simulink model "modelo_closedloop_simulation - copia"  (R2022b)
settings: Solver=ode45  StartTime=0.0  StopTime=1  MaxStep=1e-6  RelTol=1e-3
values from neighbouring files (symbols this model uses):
  fsw = 36e3    (= 36000)    [closedloop_analysis - copia.m]
  ki = wc*R    (= 20)    [closedloop_analysis - copia.m]
  kp = wc*L    (= 0.2)    [closedloop_analysis - copia.m]
  L = 100e-6    (= 0.0001)    [closedloop_analysis - copia.m]
  R = 0.01    [closedloop_analysis - copia.m]
  Ts = Tsw    (= 2.77777777778e-05)    [closedloop_analysis - copia.m]
  Tsim = Tsw/400    (= 6.94444444444e-08)    [closedloop_analysis - copia.m]
  Vdc = 450    [closedloop_analysis - copia.m]
undefined symbols (not defined in the file or in its folder): arm, bridge, pulses
libraries: simulink x12, spsMosfetLib x6, spsCurrentMeasurementLib x3, spsSeriesRLCBranchLib x3, powerlib_extras x3, slpidlib x2, spsControlledVoltageSourceLib x1, spsGroundLib x1, spsDCVoltageSourceLib x1, sps_lib x1

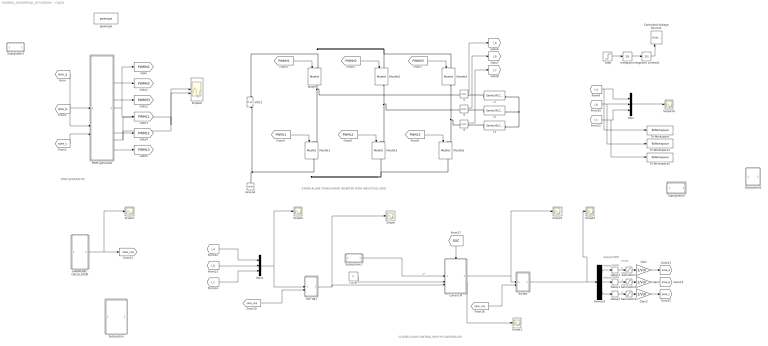
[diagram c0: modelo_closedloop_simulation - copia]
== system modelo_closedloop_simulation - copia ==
  note: CLOSED LOOP CONTROL WITH PI CONTROLLER
  note: STAND ALONE THREE-PHASE INVERTER WITH INDUCTIVE LOAD
  note: PWM GENERATOR
  note: vmax
  note: reload PWM
  note: vmax
  note: reload PWM
  note: reload PWM
  note: vmax
  Controlled Voltage Source1 : spsControlledVoltageSourceLib/Controlled Voltage Source  Commented=on  Initialize=on  Source_Type=AC  Amplitude=0  Phase=0  Frequency=0  Measurements=None
  Delay1 : Delay  DelayLength=1  SampleTime=Ts/2
  Delay2 : Delay  DelayLength=1  SampleTime=Ts/2
  Delay3 : Delay  DelayLength=1  SampleTime=Ts/2
  Demux5 : Demux  Outputs=3
  Gain : Gain  Gain=1/Vdc
  Gain1 : Gain  Gain=1/Vdc
  Gain2 : Gain  Gain=1/Vdc
  Ground : spsGroundLib/Ground  LConnTagsString=a
  HARMONIC OSCILLATOR : Subsystem
  I1 : spsCurrentMeasurementLib/Current Measurement  PhasorSimulation=off  OutputType=Complex  PSBequivalent=0
  I2 : spsCurrentMeasurementLib/Current Measurement  PhasorSimulation=off  OutputType=Complex  PSBequivalent=0
  I3 : spsCurrentMeasurementLib/Current Measurement  PhasorSimulation=off  OutputType=Complex  PSBequivalent=0
  Integrator : Integrator  Commented=on
  Integrator Limited1 : Integrator  Commented=on  LimitOutput=on  UpperSaturationLimit=900  LowerSaturationLimit=0
  L1 : spsSeriesRLCBranchLib/Series RLC Branch  LConnTagsString=__new0  RConnTagsString=__new0  BranchType=RL  Resistance=R  Inductance=L  SetiL0=off  InitialCurrent=0  Capacitance=1e-6  Setx0=off  InitialVoltage=0  Measurements=None
  L2 : spsSeriesRLCBranchLib/Series RLC Branch  LConnTagsString=__new0  RConnTagsString=__new0  BranchType=RL  Resistance=R  Inductance=L  SetiL0=off  InitialCurrent=0  Capacitance=1e-6  Setx0=off  InitialVoltage=0  Measurements=None
  L3 : spsSeriesRLCBranchLib/Series RLC Branch  LConnTagsString=__new0  RConnTagsString=__new0  BranchType=RL  Resistance=R  Inductance=L  SetiL0=off  InitialCurrent=0  Capacitance=1e-6  Setx0=off  InitialVoltage=0  Measurements=None
  Mosfet{,1..5} (6 alike) : spsMosfetLib/Mosfet  Ron=0.1  Lon=0  Rd=0.01  Vfd=1  IC=0  Rs=1e5  Cs=inf  Measurements=off
  Mux : Mux  Inputs=3
  Mux1 : Mux  Inputs=3
  PWM generator : Subsystem
  Saturation : Saturate  UpperLimit=Vdc*0.98  LowerLimit=0
  Saturation1 : Saturate  UpperLimit=Vdc*0.98  LowerLimit=0
  Saturation2 : Saturate  UpperLimit=Vdc*0.98  LowerLimit=0
  Scope{,1..3,5,7,10} (7 alike) : Scope
  Scope9 : Scope  NumInputPorts=2
  Step : Step  Commented=on  Time=0  After=2500  SampleTime=0
  Subsystem : Subsystem  Commented=on
  Subsystem1 : Subsystem
  Subsystem2 : Subsystem  Commented=on
  Subsystem3 : Subsystem  Commented=on
  Subsystem4 : Subsystem
  To Workspace : ToWorkspace  VariableName=i_a  SaveFormat=Structure With Time  SampleTime=-1
  To Workspace1 : ToWorkspace  VariableName=i_b  SaveFormat=Structure With Time  SampleTime=-1
  To Workspace2 : ToWorkspace  VariableName=i_c  SaveFormat=Structure With Time  SampleTime=-1
  VDC1 : spsDCVoltageSourceLib/DC Voltage Source  Amplitude=Vdc*2  Measurements=None
  abc-dq1 : Subsystem
  current PI : Subsystem
  dq-abc : Subsystem
  i_q ref : Constant  Value=0
  powergui : sps_lib/powergui  Priority=1  SimulationMode=Continuous  SampleTime=50e-6  frequency=60  Iterations=50  frequencyindice=0  Pbase=100e6  ErrMax=1e-4  UnitsV=kV  UnitsW=MW  buscounter=0  FunctionMessages=off  echomessages=off  EnableUseOfTLC=off  CurrentSourceSwitches=off  DisableSnubberDevices=off  DisableRonSwitches=off  DisableVfSwitches=off  DisplayEquations=off  AutomaticDiscreteSolvers=off  SolverType=Tustin/Backward Euler (TBE)  Interpol=off  ExternalGateDelay=off  methode=off  Ts=100  x0status=blocks  SPID=on  SwTol=0  HookPort=off  NonlinearTolerance=1e-4  nMaxIteration=100  ContinueOnMaxIteration=off  RestoreLinks=warning  ResistiveCurrentMeasurement=off  Frange=[0:2:500]  Ylog=off  Xlog=on  ShowGrid=off  save=off  variable=ZData  structure=0  ZoomFFT=off  StartTime=0.0  cycles=1  DisplayStyle=1  fundamental=60  FreqAxis=off  MaxFrequency=1000  frequencyindicesteady=1  RmsSteady=1  display=off
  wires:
  [sine_a] -> PWM generator/1(m1)
  [sine_b] -> PWM generator/2(m2)
  [sine_c] -> PWM generator/3(m3)
  PWM generator/1(PWMH1) -> Scope9/1, [PWMH1]
  PWM generator/2(PWMH2) -> [PWMH2]
  PWM generator/3(PWMH3) -> [PWMH3]
  PWM generator/4(PWML1) -> Scope9/2, [PWML1]
  PWM generator/5(PWML2) -> [PWML2]
  PWM generator/6(PWML3) -> [PWML3]
  [PWMH1] -> Mosfet/1
  [PWML1] -> Mosfet1/1
  [PWML2] -> Mosfet3/1
  [PWMH2] -> Mosfet2/1
  [PWML3] -> Mosfet5/1
  [PWMH3] -> Mosfet4/1
  I1/1 -> [i_a]
  I2/1 -> [i_b]
  I3/1 -> [i_c]
  HARMONIC OSCILLATOR/1(sin-cos) -> Scope7/1, [sine_cos]
  [i_c] -> Mux1/3
  [i_b] -> Mux1/2
  [i_a] -> Mux1/1
  Mux1/1 -> Scope5/1, abc-dq1/1(abc)
  [sine_cos] -> abc-dq1/2(sin-cos)
  abc-dq1/1(dq) -> Scope/1, current PI/3(dq pi in)
  [sine_cos] -> dq-abc/2(sin-cos)
  Step/1 -> Integrator/1
  Integrator/1 -> Integrator Limited1/1
  Integrator Limited1/1 -> Controlled Voltage Source1/1
  dq-abc/1(abc) -> Scope3/1, Demux5/1
  current PI/1(dq pi out) -> dq-abc/1(dq), Scope2/1
  [i_a] -> To Workspace/1, Mux/1
  [i_b] -> To Workspace1/1, Mux/2
  [i_c] -> To Workspace2/1, Mux/3
  Mux/1 -> Scope10/1
  i_q ref/1 -> current PI/2(q ref)
  Subsystem1/1(y*) -> current PI/1(d ref)  "y*"
  Delay3/1 -> Saturation/1  "u"
  Saturation/1 -> Gain/1
  Delay1/1 -> Saturation1/1  "u"
  Saturation1/1 -> Gain1/1
  Delay2/1 -> Saturation2/1  "u"
  Saturation2/1 -> Gain2/1
  Demux5/3 -> Delay2/1
  Demux5/2 -> Delay1/1
  Demux5/1 -> Delay3/1
  Gain/1 -> [sine_a]
  Gain1/1 -> [sine_b]
  Gain2/1 -> [sine_c]
  [SOC] -> current PI/Trigger
  current PI/2(debug) -> Scope1/1
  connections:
  Mosfet/RConn1 -- I1/LConn1 -- Mosfet1/LConn1
  Mosfet2/RConn1 -- I2/LConn1 -- Mosfet3/LConn1
  L3/LConn1 -- I3/RConn1
  VDC1/RConn1 -- Mosfet4/LConn1 -- Mosfet2/LConn1 -- Mosfet/LConn1
  Mosfet1/RConn1 -- Mosfet3/RConn1 -- Mosfet5/RConn1 -- Ground/LConn1 -- VDC1/LConn1
  L1/RConn1 -- L2/RConn1 -- L3/RConn1
  L1/LConn1 -- I1/RConn1
  L2/LConn1 -- I2/RConn1
  Mosfet4/RConn1 -- I3/LConn1 -- Mosfet5/LConn1

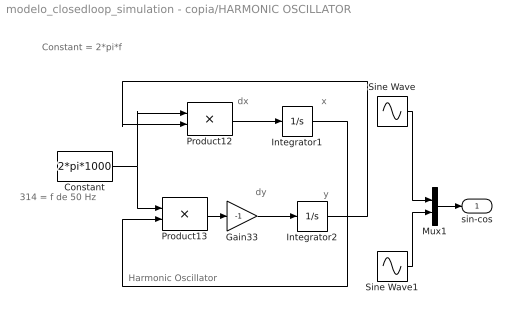
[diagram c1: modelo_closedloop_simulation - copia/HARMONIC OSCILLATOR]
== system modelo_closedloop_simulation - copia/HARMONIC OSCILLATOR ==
  note: 314 = f de 50 Hz
  note: Constant = 2*pi*f
  note: Harmonic Oscillator
  note: dy
  note: dx
  note: y
  note: x
  Constant : Constant  Commented=on  Value=2*pi*1000
  Gain33 : Gain  Commented=on  Gain=-1  SaturateOnIntegerOverflow=on
  Integrator1 : Integrator  Commented=on  InitialCondition=1  LimitOutput=on  UpperSaturationLimit=1  LowerSaturationLimit=-1
  Integrator2 : Integrator  Commented=on  LimitOutput=on  UpperSaturationLimit=1  LowerSaturationLimit=-1
  Mux1 : Mux  Inputs=2
  Product12 : Product  Commented=on  SaturateOnIntegerOverflow=on
  Product13 : Product  Commented=on  SaturateOnIntegerOverflow=on
  Sine Wave : Sin  SineType=Sample based  Samples=fsw/1000  SampleTime=Ts
  Sine Wave1 : Sin  SineType=Sample based  Samples=fsw/1000  SampleTime=Ts
  sin-cos : Outport  VectorParamsAs1DForOutWhenUnconnected=off
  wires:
  Constant/1 -> Product13/1, Product12/1
  Gain33/1 -> Integrator2/1
  Product12/1 -> Integrator1/1
  Product13/1 -> Gain33/1
  Integrator1/1 -> Product13/2
  Integrator2/1 -> Product12/2
  Mux1/1 -> sin-cos/1
  Sine Wave1/1 -> Mux1/2
  Sine Wave/1 -> Mux1/1

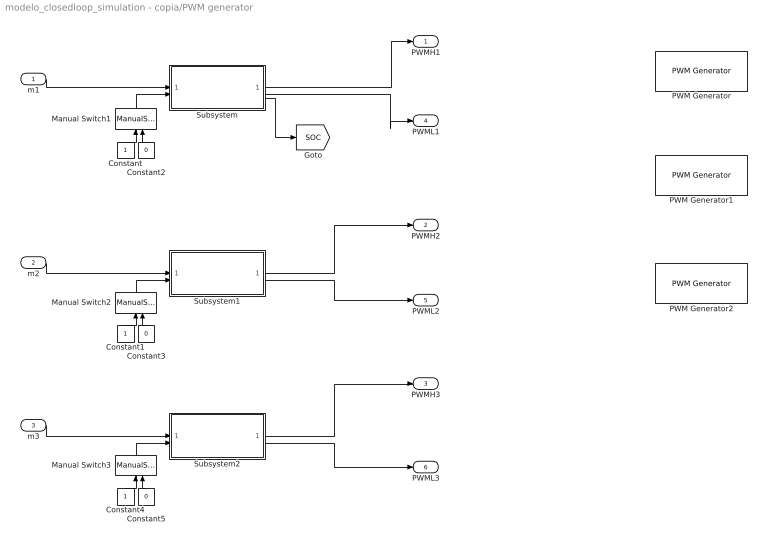
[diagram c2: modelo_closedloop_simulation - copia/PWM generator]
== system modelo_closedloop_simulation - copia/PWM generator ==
  m1 : Inport
  m2 : Inport  Port=2
  m3 : Inport  Port=3
  Constant : Constant  SampleTime=Ts
  Constant1 : Constant  SampleTime=Ts
  Constant2 : Constant  Value=0  SampleTime=Ts
  Constant3 : Constant  Value=0  SampleTime=Ts
  Constant4 : Constant  SampleTime=Ts
  Constant5 : Constant  Value=0  SampleTime=Ts
  Manual Switch1 : ManualSwitch
  Manual Switch2 : ManualSwitch
  Manual Switch3 : ManualSwitch
  PWM Generator : powerlib_extras/Control  Blocks/PWM Generator  Commented=on  GeneratorMode="1-arm  bridge (2 pulses)"  Fc=36e3  Internal=off  mIndex=0.4  Freq=60  Phase=0
  PWM Generator1 : powerlib_extras/Control  Blocks/PWM Generator  Commented=on  GeneratorMode="1-arm  bridge (2 pulses)"  Fc=36e3  Internal=off  mIndex=0.4  Freq=60  Phase=0
  PWM Generator2 : powerlib_extras/Control  Blocks/PWM Generator  Commented=on  GeneratorMode="1-arm  bridge (2 pulses)"  Fc=36e3  Internal=off  mIndex=0.4  Freq=60  Phase=0
  Subsystem : Subsystem
  Subsystem1 : Subsystem
  Subsystem2 : Subsystem
  PWMH1 : Outport  VectorParamsAs1DForOutWhenUnconnected=off
  PWMH2 : Outport  Port=2  VectorParamsAs1DForOutWhenUnconnected=off
  PWMH3 : Outport  Port=3  VectorParamsAs1DForOutWhenUnconnected=off
  PWML1 : Outport  Port=4  VectorParamsAs1DForOutWhenUnconnected=off
  PWML2 : Outport  Port=5  VectorParamsAs1DForOutWhenUnconnected=off
  PWML3 : Outport  Port=6  VectorParamsAs1DForOutWhenUnconnected=off
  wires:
  Subsystem1/2(s1B) -> PWML2/1
  Subsystem/2(s1B) -> PWML1/1
  Subsystem/1(s1A) -> PWMH1/1
  Subsystem/3(SOC) -> [SOC]
  m1/1 -> Subsystem/1(modA)
  Constant/1 -> Manual Switch1/1
  Constant2/1 -> Manual Switch1/2
  Manual Switch1/1 -> Subsystem/2(enable delay)
  Manual Switch2/1 -> Subsystem1/2(enable delay)
  Constant3/1 -> Manual Switch2/2
  Constant1/1 -> Manual Switch2/1
  m2/1 -> Subsystem1/1(modA)
  Subsystem1/1(s1A) -> PWMH2/1
  Manual Switch3/1 -> Subsystem2/2(enable delay)
  Constant5/1 -> Manual Switch3/2
  Subsystem2/2(s1B) -> PWML3/1
  Constant4/1 -> Manual Switch3/1
  m3/1 -> Subsystem2/1(modA)
  Subsystem2/1(s1A) -> PWMH3/1

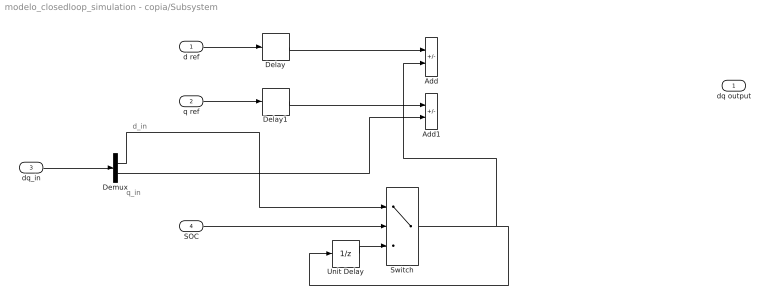
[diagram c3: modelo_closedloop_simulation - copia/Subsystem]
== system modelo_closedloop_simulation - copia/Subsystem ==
  note: q_in
  note: d_in
  d ref : Inport
  q ref : Inport  Port=2
  dq_in : Inport  Port=3
  SOC : Inport  Port=4
  Add : Sum  Inputs=+-
  Add1 : Sum  Inputs=+-
  Delay : Delay  DelayLength=1  SampleTime=Ts/2
  Delay1 : Delay  DelayLength=1  SampleTime=Ts/2
  Demux : Demux  Outputs=2
  Switch : Switch
  Unit Delay : UnitDelay  SampleTime=-1  HasFrameUpgradeWarning=on
  dq output : Outport
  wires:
  d ref/1 -> Delay/1
  q ref/1 -> Delay1/1
  dq_in/1 -> Demux/1
  Demux/1 -> Switch/1
  Delay/1 -> Add/1
  Demux/2 -> Add1/2
  Delay1/1 -> Add1/1
  SOC/1 -> Switch/2
  Unit Delay/1 -> Switch/3
  Switch/1 -> Add/2, Unit Delay/1

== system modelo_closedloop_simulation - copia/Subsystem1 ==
  note: in practice period of 1.352s
  Add2 : Sum
  Constant : Constant  Value=127.3
  Pulse Generator : DiscretePulseGenerator  PulseType=Time based  Amplitude=6  Period=3  PulseWidth=50
  pulses : DiscretePulseGenerator  Amplitude=127.3  Period=120  PulseWidth=60  PhaseDelay=5  SampleTime=Ts
  reference step : Step  Time=2e-3  After=1.8  SampleTime=Ts
  reference step1 : Step  Time=0.01  After=-1.8  SampleTime=Ts
  y* : Outport  VectorParamsAs1DForOutWhenUnconnected=off
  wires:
  reference step1/1 -> Add2/2  "y2"
  pulses/1 -> y*/1, [iref]  "y*"
  reference step/1 -> Add2/1  "y1"

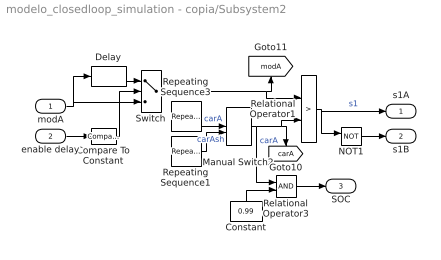
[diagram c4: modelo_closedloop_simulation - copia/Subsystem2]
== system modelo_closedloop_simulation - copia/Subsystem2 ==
  modA : Inport
  enable delay : Inport  Port=2
  Compare To Constant : simulink/Logic and Bit Operations/Compare To Constant  relop=>  const=0  OutDataTypeStr=boolean
  Constant : Constant  Value=0.99  SampleTime=Ts
  Delay : Delay  DelayLength=400  SampleTime=Tsim
  Manual Switch2 : ManualSwitch
  NOT1 : Logic  Operator=NOT  IconShape=distinctive  AllPortsSameDT=off  OutDataTypeStr=boolean
  Relational Operator1 : RelationalOperator  Operator=>  OutDataTypeStr=boolean  RndMeth=Simplest
  Relational Operator3 : RelationalOperator  OutDataTypeStr=boolean  RndMeth=Simplest
  Repeating Sequence1 : simulink/Sources/Repeating Sequence  rep_seq_t=[0 1/(4*fsw) 1/(2*fsw) 3/(4*fsw) 1/fsw]  rep_seq_y=[0.5 0 0.5 1 0.5]
  Repeating Sequence3 : simulink/Sources/Repeating Sequence  rep_seq_t=[0 1/(2*fsw) 1/fsw]  rep_seq_y=[0 1 0]
  Switch : Switch  Criteria=u2 > Threshold
  s1A : Outport  VectorParamsAs1DForOutWhenUnconnected=off
  s1B : Outport  Port=2  VectorParamsAs1DForOutWhenUnconnected=off
  SOC : Outport  Port=3  VectorParamsAs1DForOutWhenUnconnected=off
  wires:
  enable delay/1 -> Compare To Constant/1
  Relational Operator1/1 -> NOT1/1, s1A/1  "s1"
  Relational Operator3/1 -> SOC/1
  NOT1/1 -> s1B/1
  Constant/1 -> Relational Operator3/2
  Switch/1 -> Relational Operator1/1, [modA]
  modA/1 -> Delay/1, Switch/3
  Repeating Sequence1/1 -> Manual Switch2/2  "carAsh"
  Delay/1 -> Switch/1
  Manual Switch2/1 -> Relational Operator3/1, [carA], Relational Operator1/2  "carA"
  Repeating Sequence3/1 -> Manual Switch2/1  "carA"
  Compare To Constant/1 -> Switch/2

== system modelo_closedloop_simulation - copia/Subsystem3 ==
  note: in practice period of 1.352s
  Add2 : Sum
  Pulse Generator : DiscretePulseGenerator  PulseType=Time based  Amplitude=6  Period=3  PulseWidth=50
  pulses : DiscretePulseGenerator  Amplitude=1.5  Period=120  PulseWidth=60  PhaseDelay=5  SampleTime=Ts
  reference step : Step  Time=2e-3  After=1.8  SampleTime=Ts
  reference step1 : Step  Time=0.01  After=-1.8  SampleTime=Ts
  y* : Outport  VectorParamsAs1DForOutWhenUnconnected=off
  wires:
  reference step1/1 -> Add2/2  "y2"
  pulses/1 -> [iref], y*/1  "y*"
  reference step/1 -> Add2/1  "y1"

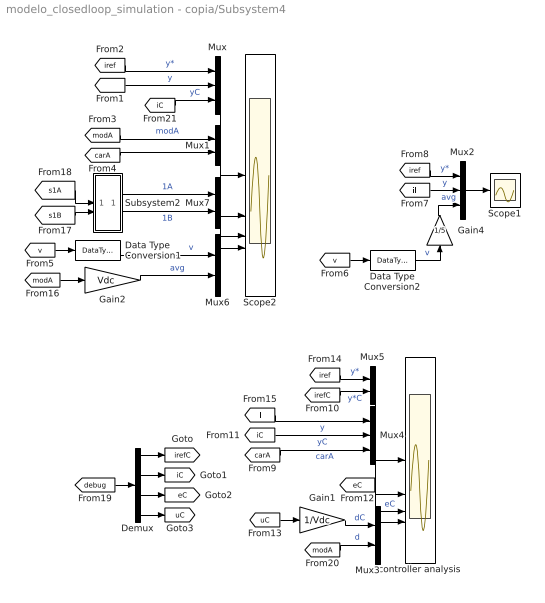
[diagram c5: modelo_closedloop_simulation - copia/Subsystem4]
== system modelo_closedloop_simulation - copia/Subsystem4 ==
  Data Type Conversion1 : DataTypeConversion  OutDataTypeStr=double
  Data Type Conversion2 : DataTypeConversion  OutDataTypeStr=double
  Demux : Demux
  Gain1 : Gain  Gain=1/Vdc
  Gain2 : Gain  Gain=Vdc
  Gain4 : Gain  Gain=1/5
  Mux : Mux  Inputs=3
  Mux{1,3,5..7} (5 alike) : Mux  Inputs=2
  Mux2 : Mux  Inputs=3
  Mux4 : Mux  Inputs=3
  Scope1 : Scope
  Scope2 : Scope  NumInputPorts=4
  Subsystem2 : Subsystem
  controller analysis : Scope  NumInputPorts=4
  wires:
  Mux1/1 -> Scope2/2
  Data Type Conversion1/1 -> Mux6/1  "v"
  [modA] -> Gain2/1
  Mux6/1 -> Scope2/4
  [carA] -> Mux1/2
  [v] -> Data Type Conversion1/1
  [s1B] -> Subsystem2/2(In2)
  Gain2/1 -> Mux6/2  "avg"
  Subsystem2/1(Out1) -> Mux7/1  "1A"
  Mux7/1 -> Scope2/3
  [modA] -> Mux1/1  "modA"
  Subsystem2/2(Out2) -> Mux7/2  "1B"
  [s1A] -> Subsystem2/1(In1)
  [v] -> Data Type Conversion2/1
  Data Type Conversion2/1 -> Gain4/1  "v"
  [iref] -> Mux2/1  "y*"
  [il] -> Mux2/2  "y"
  Mux2/1 -> Scope1/1
  Gain4/1 -> Mux2/3  "avg"
  [iref] -> Mux/1  "y*"
  [il] -> Mux/2  "y"
  Mux/1 -> Scope2/1
  [eC] -> controller analysis/3  "eC"
  Mux3/1 -> controller analysis/4
  Mux5/1 -> controller analysis/1
  Mux4/1 -> controller analysis/2
  [iref] -> Mux5/1  "y*"
  [uC] -> Gain1/1
  [il] -> Mux4/1  "y"
  [iC] -> Mux4/2  "yC"
  [carA] -> Mux4/3  "carA"
  [modA] -> Mux3/2  "d"
  [debug] -> Demux/1
  Demux/3 -> [eC]
  Demux/2 -> [iC]
  Demux/1 -> [irefC]
  Demux/4 -> [uC]
  [irefC] -> Mux5/2  "y*C"
  Gain1/1 -> Mux3/1  "dC"
  [iC] -> Mux/3  "yC"

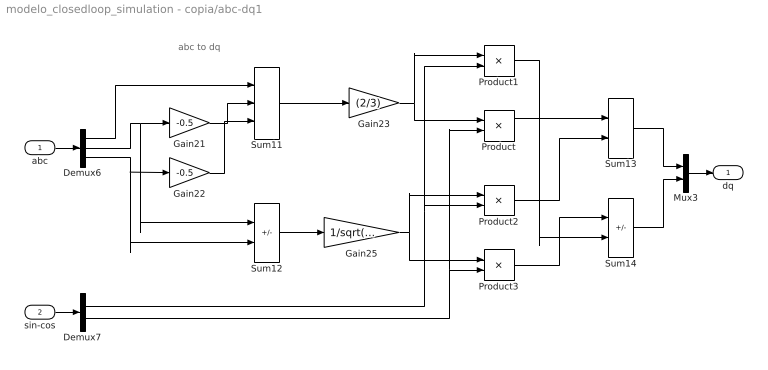
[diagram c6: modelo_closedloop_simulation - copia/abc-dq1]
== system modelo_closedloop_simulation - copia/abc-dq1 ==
  note: abc to dq
  abc : Inport
  sin-cos : Inport  Port=2
  Demux6 : Demux  Outputs=3
  Demux7 : Demux  Outputs=2
  Gain21 : Gain  Gain=-0.5
  Gain22 : Gain  Gain=-0.5
  Gain23 : Gain  Gain=(2/3)
  Gain25 : Gain  Gain=1/sqrt(3)
  Mux3 : Mux  Inputs=2
  Product{,1..3} (4 alike) : Product  RndMeth=Zero
  Sum11 : Sum  Inputs=|+++
  Sum12 : Sum  Inputs=|+-
  Sum13 : Sum  Inputs=|++
  Sum14 : Sum  Inputs=|+-
  dq : Outport  VectorParamsAs1DForOutWhenUnconnected=off
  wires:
  Sum11/1 -> Gain23/1
  Sum12/1 -> Gain25/1
  Demux6/3 -> Gain22/1, Sum12/2
  Demux6/2 -> Gain21/1, Sum12/1
  Demux6/1 -> Sum11/1
  Gain21/1 -> Sum11/2
  Gain22/1 -> Sum11/3
  Gain23/1 -> Product/1, Product1/1
  Demux7/2 -> Product/2, Product3/2
  Demux7/1 -> Product1/2, Product2/2
  Gain25/1 -> Product2/1, Product3/1
  Product/1 -> Sum13/1
  Product2/1 -> Sum13/2
  Product3/1 -> Sum14/1
  Product1/1 -> Sum14/2
  Sum13/1 -> Mux3/1
  Sum14/1 -> Mux3/2
  abc/1 -> Demux6/1
  Mux3/1 -> dq/1
  sin-cos/1 -> Demux7/1

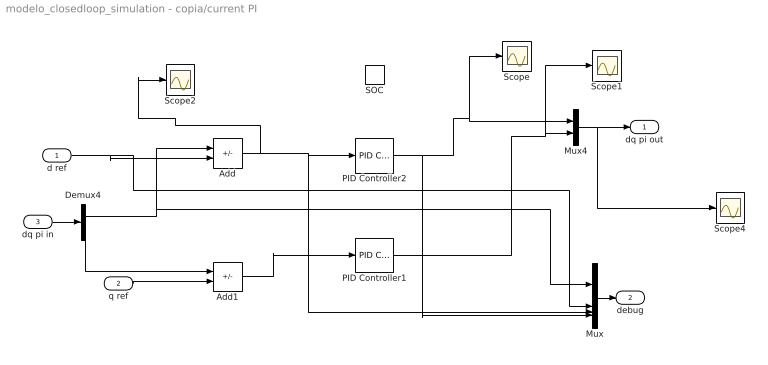
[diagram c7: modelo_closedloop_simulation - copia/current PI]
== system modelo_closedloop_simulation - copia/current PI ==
  d ref : Inport
  q ref : Inport  Port=2
  dq pi in : Inport  Port=3
  SOC : TriggerPort  VariantControl=Variant
  Add : Sum  Inputs=+-
  Add1 : Sum  Inputs=+-
  Demux4 : Demux  Outputs=2
  Mux : Mux
  Mux4 : Mux  Inputs=2
  PID Controller1 : slpidlib/PID Controller  Controller=PI  Form=Parallel  TimeDomain=Discrete-time  UseExternalTs=off  SampleTime=-1  IntegratorMethod=Backward Euler  FilterMethod=Forward Euler  ControllerParametersSource=internal  P=kp  I=ki  UseKiTs=off  D=0  N=100  UseFilter=on  TunerSelectOption=Transfer Function Based (PID Tuner App)  InitialConditionSource=internal  InitialConditionForIntegrator=0  InitialConditionForFilter=0  DifferentiatorICPrevScaledInput=0  ExternalReset=none  TrackingMode=off  Kt=1  LimitOutput=off  SatLimitsSource=internal  UpperSaturationLimit=Vdc*0.98  LowerSaturationLimit=0  LinearizeAsGain=on  AntiWindupMode=back-calculation  Kb=ki/kp  LimitIntegrator=off  UpperIntegratorSaturationLimit=inf  LowerIntegratorSaturationLimit=-inf  POutMin=[]  POutMax=[]  IOutMin=[]  IOutMax=[]  DOutMin=[]  DOutMax=[]  NOutMin=[]  NOutMax=[]  SumOutMin=[]  SumOutMax=[]  SaturationOutMin=[]  SaturationOutMax=[]  PParamMin=[]  PParamMax=[]  IParamMin=[]  IParamMax=[]  DParamMin=[]  DParamMax=[]  NParamMin=[]  NParamMax=[]  KbParamMin=[]  KbParamMax=[]  KtParamMin=[]  KtParamMax=[]  KbOutMin=[]  KbOutMax=[]  KtOutMin=[]  KtOutMax=[]  IntegratorOutMin=[]  IntegratorOutMax=[]  FilterOutMin=[]  FilterOutMax=[]  SumI1OutMin=[]  SumI1OutMax=[]  SumI2OutMin=[]  SumI2OutMax=[]  SumI3OutMin=[]  SumI3OutMax=[]  SumI4OutMin=[]  SumI4OutMax=[]  SumDOutMin=[]  SumDOutMax=[]  DifferentiatorOutMin=[]  DifferentiatorOutMax=[]  FilterDiffOutCoefMin=[]  FilterDiffOutCoefMax=[]  ReciprocalOutMin=[]  ReciprocalOutMax=[]  SumDenOutMin=[]  SumDenOutMax=[]  SumNumOutMin=[]  SumNumOutMax=[]  DivideOutMin=[]  DivideOutMax=[]  UdiffTsProdOutMin=[]  UdiffTsProdOutMax=[]  NTsProdOutMin=[]  NTsProdOutMax=[]  UintegralTsProdOutMin=[]  UintegralTsProdOutMax=[]  UngainTsProdOutMin=[]  UngainTsProdOutMax=[]  ClampingZeroOutDataTypeStr=Inherit: Inherit via back propagation  ClampingZeroOutMin=[]  ClampingZeroOutMax=[]  FilterDenConstantOutDataTypeStr=Inherit: Inherit via back propagation  FilterDenConstantOutMin=[]  FilterDenConstantOutMax=[]  PCopyOutDataTypeStr=Inherit: Inherit via back propagation  PCopyOutMin=[]  PCopyOutMax=[]  NCopyOutDataTypeStr=Inherit: Inherit via back propagation  NCopyOutMin=[]  NCopyOutMax=[]  IntegratorContinuousStateAttributes=''  IntegratorStateMustResolveToSignalObject=off  IntegratorRTWStateStorageClass=Auto  FilterContinuousStateAttributes=''  FilterStateMustResolveToSignalObject=off  FilterRTWStateStorageClass=Auto  ParallelPVariant=InternalParameters  IdealPVariant=Disabled  IVariant=InternalParameters  DVariant=Disabled  IntegratorVariant=Discrete  SatVariant=Disabled  AWVariant=Passthrough  PCopyVariant=Disabled  TRVariant=Disabled  FdbkBlocksVariant=Forward  IdealPFdbkVariant=Disabled  SatFdbkVariant=Disabled  DerivativeFilterVariant=Disabled  NVariant=Disabled  NCopyVariant=Disabled_SignalSpec  FilterICVariant=Disabled  IntegratorICVariant=InternalICs  ExternalResetVariant=Disabled  TRSumVariant=Passthrough  SumFdbkVariant=Disabled  SumVariant=Sum_PI  TsampFilterVariant=InternalTs  TsampNgainVariant=Passthrough  TsampIntegralVariant=Passthrough  ExternalSaturationOutDataTypeStr=Inherit: Same as second input
  PID Controller2 : slpidlib/PID Controller  Controller=PI  Form=Parallel  TimeDomain=Discrete-time  UseExternalTs=off  SampleTime=-1  IntegratorMethod=Backward Euler  FilterMethod=Forward Euler  ControllerParametersSource=internal  P=kp  I=ki  UseKiTs=off  D=0  N=100  UseFilter=on  TunerSelectOption=Transfer Function Based (PID Tuner App)  InitialConditionSource=internal  InitialConditionForIntegrator=0  InitialConditionForFilter=0  DifferentiatorICPrevScaledInput=0  ExternalReset=none  TrackingMode=off  Kt=1  LimitOutput=off  SatLimitsSource=internal  UpperSaturationLimit=Vdc*0.98  LowerSaturationLimit=0  LinearizeAsGain=on  AntiWindupMode=back-calculation  Kb=ki/kp  LimitIntegrator=off  UpperIntegratorSaturationLimit=inf  LowerIntegratorSaturationLimit=-inf  POutMin=[]  POutMax=[]  IOutMin=[]  IOutMax=[]  DOutMin=[]  DOutMax=[]  NOutMin=[]  NOutMax=[]  SumOutMin=[]  SumOutMax=[]  SaturationOutMin=[]  SaturationOutMax=[]  PParamMin=[]  PParamMax=[]  IParamMin=[]  IParamMax=[]  DParamMin=[]  DParamMax=[]  NParamMin=[]  NParamMax=[]  KbParamMin=[]  KbParamMax=[]  KtParamMin=[]  KtParamMax=[]  KbOutMin=[]  KbOutMax=[]  KtOutMin=[]  KtOutMax=[]  IntegratorOutMin=[]  IntegratorOutMax=[]  FilterOutMin=[]  FilterOutMax=[]  SumI1OutMin=[]  SumI1OutMax=[]  SumI2OutMin=[]  SumI2OutMax=[]  SumI3OutMin=[]  SumI3OutMax=[]  SumI4OutMin=[]  SumI4OutMax=[]  SumDOutMin=[]  SumDOutMax=[]  DifferentiatorOutMin=[]  DifferentiatorOutMax=[]  FilterDiffOutCoefMin=[]  FilterDiffOutCoefMax=[]  ReciprocalOutMin=[]  ReciprocalOutMax=[]  SumDenOutMin=[]  SumDenOutMax=[]  SumNumOutMin=[]  SumNumOutMax=[]  DivideOutMin=[]  DivideOutMax=[]  UdiffTsProdOutMin=[]  UdiffTsProdOutMax=[]  NTsProdOutMin=[]  NTsProdOutMax=[]  UintegralTsProdOutMin=[]  UintegralTsProdOutMax=[]  UngainTsProdOutMin=[]  UngainTsProdOutMax=[]  ClampingZeroOutDataTypeStr=Inherit: Inherit via back propagation  ClampingZeroOutMin=[]  ClampingZeroOutMax=[]  FilterDenConstantOutDataTypeStr=Inherit: Inherit via back propagation  FilterDenConstantOutMin=[]  FilterDenConstantOutMax=[]  PCopyOutDataTypeStr=Inherit: Inherit via back propagation  PCopyOutMin=[]  PCopyOutMax=[]  NCopyOutDataTypeStr=Inherit: Inherit via back propagation  NCopyOutMin=[]  NCopyOutMax=[]  IntegratorContinuousStateAttributes=''  IntegratorStateMustResolveToSignalObject=off  IntegratorRTWStateStorageClass=Auto  FilterContinuousStateAttributes=''  FilterStateMustResolveToSignalObject=off  FilterRTWStateStorageClass=Auto  ParallelPVariant=InternalParameters  IdealPVariant=Disabled  IVariant=InternalParameters  DVariant=Disabled  IntegratorVariant=Discrete  SatVariant=Disabled  AWVariant=Passthrough  PCopyVariant=Disabled  TRVariant=Disabled  FdbkBlocksVariant=Forward  IdealPFdbkVariant=Disabled  SatFdbkVariant=Disabled  DerivativeFilterVariant=Disabled  NVariant=Disabled  NCopyVariant=Disabled_SignalSpec  FilterICVariant=Disabled  IntegratorICVariant=InternalICs  ExternalResetVariant=Disabled  TRSumVariant=Passthrough  SumFdbkVariant=Disabled  SumVariant=Sum_PI  TsampFilterVariant=InternalTs  TsampNgainVariant=Passthrough  TsampIntegralVariant=Passthrough  ExternalSaturationOutDataTypeStr=Inherit: Same as second input
  Scope{,1..2,4} (4 alike) : Scope
  dq pi out : Outport  VectorParamsAs1DForOutWhenUnconnected=off
  debug : Outport  Port=2  VectorParamsAs1DForOutWhenUnconnected=off
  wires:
  Add/1 -> Mux/3, PID Controller2/1, Scope2/1
  Mux4/1 -> Scope4/1, dq pi out/1
  dq pi in/1 -> Demux4/1
  q ref/1 -> Add1/2
  Demux4/1 -> Add/1, Mux/1
  Demux4/2 -> Add1/1
  PID Controller1/1 -> Scope1/1, Mux4/2
  Mux/1 -> debug/1
  PID Controller2/1 -> Mux/4, Scope/1, Mux4/1
  d ref/1 -> Mux/2, Add/2
  Add1/1 -> PID Controller1/1

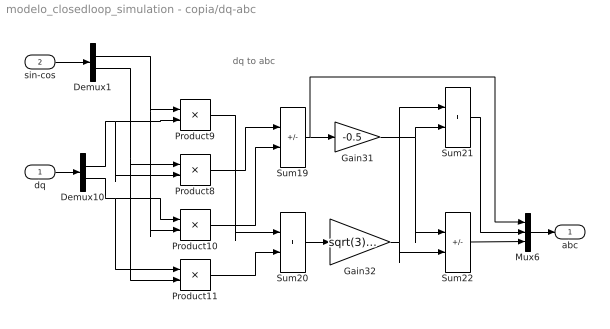
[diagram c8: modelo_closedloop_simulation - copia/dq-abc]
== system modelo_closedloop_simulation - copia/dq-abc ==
  note: dq to abc
  dq : Inport
  sin-cos : Inport  Port=2
  Demux1 : Demux  Outputs=2
  Demux10 : Demux  Outputs=2
  Gain31 : Gain  Gain=-0.5
  Gain32 : Gain  Gain=sqrt(3)/2
  Mux6 : Mux  Inputs=3
  Product{8..11} (4 alike) : Product  RndMeth=Zero
  Sum19 : Sum  Inputs=|+-
  Sum20 : Sum  Inputs=|++
  Sum21 : Sum  Inputs=|++
  Sum22 : Sum  Inputs=|+-
  abc : Outport  VectorParamsAs1DForOutWhenUnconnected=off
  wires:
  Sum22/1 -> Mux6/3
  Sum21/1 -> Mux6/2
  Demux10/2 -> Product10/1, Product11/1
  Demux10/1 -> Product9/2, Product8/2
  Gain31/1 -> Sum21/2, Sum22/1
  Gain32/1 -> Sum21/1, Sum22/2
  Sum19/1 -> Gain31/1, Mux6/1
  Sum20/1 -> Gain32/1
  Product10/1 -> Sum19/2
  Product11/1 -> Sum20/2
  Product9/1 -> Sum20/1
  Product8/1 -> Sum19/1
  Demux1/1 -> Product10/2, Product9/1
  Demux1/2 -> Product11/2, Product8/1
  dq/1 -> Demux10/1
  Mux6/1 -> abc/1
  sin-cos/1 -> Demux1/1

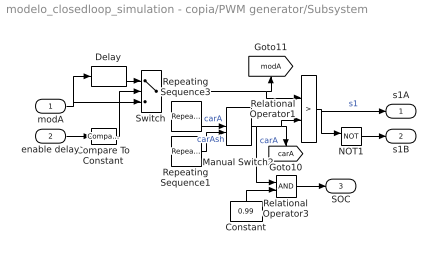
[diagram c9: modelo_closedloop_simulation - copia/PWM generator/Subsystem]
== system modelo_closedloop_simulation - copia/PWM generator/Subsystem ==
  modA : Inport
  enable delay : Inport  Port=2
  Compare To Constant : simulink/Logic and Bit Operations/Compare To Constant  relop=>  const=0  OutDataTypeStr=boolean
  Constant : Constant  Value=0.99  SampleTime=Ts
  Delay : Delay  DelayLength=400  SampleTime=Tsim
  Manual Switch2 : ManualSwitch
  NOT1 : Logic  Operator=NOT  IconShape=distinctive  AllPortsSameDT=off  OutDataTypeStr=boolean
  Relational Operator1 : RelationalOperator  Operator=>  OutDataTypeStr=boolean  RndMeth=Simplest
  Relational Operator3 : RelationalOperator  OutDataTypeStr=boolean  RndMeth=Simplest
  Repeating Sequence1 : simulink/Sources/Repeating Sequence  rep_seq_t=[0 1/(4*fsw) 1/(2*fsw) 3/(4*fsw) 1/fsw]  rep_seq_y=[0.5 0 0.5 1 0.5]
  Repeating Sequence3 : simulink/Sources/Repeating Sequence  rep_seq_t=[0 1/(2*fsw) 1/fsw]  rep_seq_y=[0 1 0]
  Switch : Switch  Criteria=u2 > Threshold
  s1A : Outport  VectorParamsAs1DForOutWhenUnconnected=off
  s1B : Outport  Port=2  VectorParamsAs1DForOutWhenUnconnected=off
  SOC : Outport  Port=3  VectorParamsAs1DForOutWhenUnconnected=off
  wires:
  enable delay/1 -> Compare To Constant/1
  Relational Operator1/1 -> NOT1/1, s1A/1  "s1"
  Relational Operator3/1 -> SOC/1
  NOT1/1 -> s1B/1
  Constant/1 -> Relational Operator3/2
  Switch/1 -> Relational Operator1/1, [modA]
  modA/1 -> Delay/1, Switch/3
  Repeating Sequence1/1 -> Manual Switch2/2  "carAsh"
  Delay/1 -> Switch/1
  Manual Switch2/1 -> Relational Operator3/1, [carA], Relational Operator1/2  "carA"
  Repeating Sequence3/1 -> Manual Switch2/1  "carA"
  Compare To Constant/1 -> Switch/2

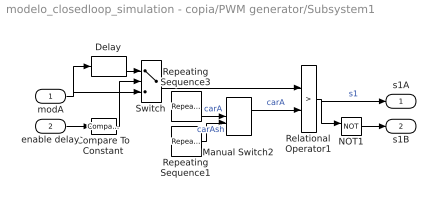
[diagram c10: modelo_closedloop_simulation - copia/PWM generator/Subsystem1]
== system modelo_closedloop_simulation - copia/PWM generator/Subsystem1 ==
  modA : Inport
  enable delay : Inport  Port=2
  Compare To Constant : simulink/Logic and Bit Operations/Compare To Constant  relop=>  const=0  OutDataTypeStr=boolean
  Delay : Delay  DelayLength=400  SampleTime=Tsim
  Manual Switch2 : ManualSwitch
  NOT1 : Logic  Operator=NOT  IconShape=distinctive  AllPortsSameDT=off  OutDataTypeStr=boolean
  Relational Operator1 : RelationalOperator  Operator=>  OutDataTypeStr=boolean  RndMeth=Simplest
  Repeating Sequence1 : simulink/Sources/Repeating Sequence  rep_seq_t=[0 1/(4*fsw) 1/(2*fsw) 3/(4*fsw) 1/fsw]  rep_seq_y=[0.5 0 0.5 1 0.5]
  Repeating Sequence3 : simulink/Sources/Repeating Sequence  rep_seq_t=[0 1/(2*fsw) 1/fsw]  rep_seq_y=[0 1 0]
  Switch : Switch  Criteria=u2 > Threshold
  s1A : Outport  VectorParamsAs1DForOutWhenUnconnected=off
  s1B : Outport  Port=2  VectorParamsAs1DForOutWhenUnconnected=off
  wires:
  enable delay/1 -> Compare To Constant/1
  Relational Operator1/1 -> NOT1/1, s1A/1  "s1"
  NOT1/1 -> s1B/1
  Switch/1 -> Relational Operator1/1
  modA/1 -> Delay/1, Switch/3
  Repeating Sequence1/1 -> Manual Switch2/2  "carAsh"
  Delay/1 -> Switch/1
  Manual Switch2/1 -> Relational Operator1/2  "carA"
  Repeating Sequence3/1 -> Manual Switch2/1  "carA"
  Compare To Constant/1 -> Switch/2

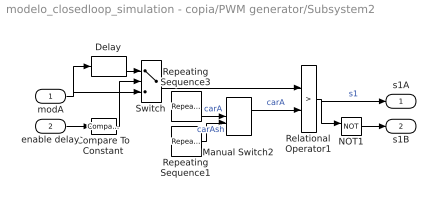
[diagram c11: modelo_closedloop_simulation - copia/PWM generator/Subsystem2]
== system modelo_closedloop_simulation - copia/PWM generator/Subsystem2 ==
  modA : Inport
  enable delay : Inport  Port=2
  Compare To Constant : simulink/Logic and Bit Operations/Compare To Constant  relop=>  const=0  OutDataTypeStr=boolean
  Delay : Delay  DelayLength=400  SampleTime=Tsim
  Manual Switch2 : ManualSwitch
  NOT1 : Logic  Operator=NOT  IconShape=distinctive  AllPortsSameDT=off  OutDataTypeStr=boolean
  Relational Operator1 : RelationalOperator  Operator=>  OutDataTypeStr=boolean  RndMeth=Simplest
  Repeating Sequence1 : simulink/Sources/Repeating Sequence  rep_seq_t=[0 1/(4*fsw) 1/(2*fsw) 3/(4*fsw) 1/fsw]  rep_seq_y=[0.5 0 0.5 1 0.5]
  Repeating Sequence3 : simulink/Sources/Repeating Sequence  rep_seq_t=[0 1/(2*fsw) 1/fsw]  rep_seq_y=[0 1 0]
  Switch : Switch  Criteria=u2 > Threshold
  s1A : Outport  VectorParamsAs1DForOutWhenUnconnected=off
  s1B : Outport  Port=2  VectorParamsAs1DForOutWhenUnconnected=off
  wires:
  enable delay/1 -> Compare To Constant/1
  Relational Operator1/1 -> NOT1/1, s1A/1  "s1"
  NOT1/1 -> s1B/1
  Switch/1 -> Relational Operator1/1
  modA/1 -> Delay/1, Switch/3
  Repeating Sequence1/1 -> Manual Switch2/2  "carAsh"
  Delay/1 -> Switch/1
  Manual Switch2/1 -> Relational Operator1/2  "carA"
  Repeating Sequence3/1 -> Manual Switch2/1  "carA"
  Compare To Constant/1 -> Switch/2

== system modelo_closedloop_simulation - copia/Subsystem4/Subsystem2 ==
  In1 : Inport
  In2 : Inport  Port=2
  Add3 : Sum
  Add4 : Sum
  Constant6 : Constant  Value=0.5  SampleTime=1/(200*fsw)
  Constant7 : Constant  Value=2  SampleTime=1/(200*fsw)
  Out1 : Outport  VectorParamsAs1DForOutWhenUnconnected=off
  Out2 : Outport  Port=2  VectorParamsAs1DForOutWhenUnconnected=off
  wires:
  In2/1 -> Add3/1
  In1/1 -> Add4/1
  Constant6/1 -> Add3/2
  Constant7/1 -> Add4/2
  Add4/1 -> Out1/1  "1A"
  Add3/1 -> Out2/1  "1B"
